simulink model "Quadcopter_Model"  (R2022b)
settings: Solver=VariableStepAuto  StartTime=0.0  StopTime=runtime  FixedStep=0.001  RelTol=1e-3
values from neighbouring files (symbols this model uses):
  delta_T = [ 0,  0,  9.404e-04 ]    [modelParameters.m]    (also in rich_params.m = [ 0,  0,  1.176e-04 ]; drone_control_system_test.m)
  g = 9.81    [modelParameters.m]    (also in rich_params.m; drone_control_system_test.m; imu_model_test.m = 0.1)
  height_controlled_o = (((Rm*If        + (((omega0_o * 2 * Rm * Kv * Kq      * Kd + 1)^2) - 1)/(4* Rm*Kv^2*Kq      * Kd))/Vb)*(Pmax - Pmin) + Pmin)    [modelParameters.m]    (also in rich_params.m)
  If = 0.3836    [modelParameters.m]    (also in rich_params.m = 0.39; drone_control_system_test.m)
  Jreq = 4.2012e-05    [modelParameters.m]    (also in rich_params.m = 1.376e-05; drone_control_system_test.m)
  Jxx = 0.0110    (= 0.011)    [modelParameters.m]    (also in rich_params.m = 0.0081; drone_control_system_test.m)
  Jyy = 0.0116    [modelParameters.m]    (also in rich_params.m = 0.0074; drone_control_system_test.m)
  Jzz = 0.0223    [modelParameters.m]    (also in rich_params.m = 0.0135; drone_control_system_test.m)
  Kd = 1.4852e-07    [modelParameters.m]    (also in rich_params.m = 5.194e-07; drone_control_system_test.m)
  Kh = 3.4574e-04    (= 0.00034574)    [modelParameters.m]    (also in rich_params.m; drone_control_system_test.m)
  Kq = 96.3422    [modelParameters.m]    (also in rich_params.m = 110; drone_control_system_test.m)
  Kt = 1.2007e-05    [modelParameters.m]    (also in rich_params.m = 7.3956e-06; drone_control_system_test.m)
  Kv = 96.3422    [modelParameters.m]    (also in rich_params.m = 110; drone_control_system_test.m)
  m = 1.216    [modelParameters.m]    (also in rich_params.m = 0.656; drone_control_system_test.m)
  omega0_o = sqrt((m*g)/(4*Kt))    [modelParameters.m]    (also in rich_params.m)
  omega1_o = sqrt((m*g)/(4*Kt))    [modelParameters.m]    (also in rich_params.m)
  omega2_o = sqrt((m*g)/(4*Kt))    [modelParameters.m]    (also in rich_params.m)
  omega3_o = sqrt((m*g)/(4*Kt))    [modelParameters.m]    (also in rich_params.m)
  pitch_o = 0    [modelParameters.m]    (also in rich_params.m)
  pitchrate_o = 0    [modelParameters.m]    (also in rich_params.m)
  Pmax = 1    [modelParameters.m]    (also in rich_params.m; drone_control_system_test.m)
  Pmin = 0    [modelParameters.m]    (also in rich_params.m; drone_control_system_test.m)
  r_oc = [ 0 ; 0 ; 0 ]    [modelParameters.m]    (also in rich_params.m; drone_control_system_test.m = [0; 0; 0]; imu_model_test.m = 0.1)
  rhx = 0.16    [modelParameters.m]    (also in rich_params.m = 0.115; drone_control_system_test.m)
  rhy = 0.16    [modelParameters.m]    (also in rich_params.m = 0.115; drone_control_system_test.m)
  rhz = 0.03    [modelParameters.m]    (also in rich_params.m = 0.04; drone_control_system_test.m)
  Rm = 0.235    [modelParameters.m]    (also in rich_params.m = 0.19; drone_control_system_test.m)
  roll_o = 0    [modelParameters.m]    (also in rich_params.m)
  rollrate_o = 0    [modelParameters.m]    (also in rich_params.m)
  signal_mixer = [ 1, -1, -1, -1    [modelParameters.m]    (also in rich_params.m; drone_control_system_test.m)
  Tc = 0.01    [modelParameters.m]    (also in rich_params.m; drone_control_system_test.m)
  Tq = 0.005    [modelParameters.m]    (also in rich_params.m; drone_control_system_test.m)
  Vb = 12.3    [modelParameters.m]    (also in rich_params.m = 11.4; drone_control_system_test.m)
  x_controlled_o = 0    [modelParameters.m]    (also in rich_params.m)
  x_o = 0    [modelParameters.m]    (also in rich_params.m)
  x_vel_o = 0    [modelParameters.m]    (also in rich_params.m)
  y_controlled_o = 0    [modelParameters.m]    (also in rich_params.m)
  y_o = 0    [modelParameters.m]    (also in rich_params.m)
  y_vel_o = 0    [modelParameters.m]    (also in rich_params.m)
  yaw_controlled_o = 0    [modelParameters.m]    (also in rich_params.m)
  yaw_o = 0    [modelParameters.m]    (also in rich_params.m)
  yawrate_o = 0    [modelParameters.m]    (also in rich_params.m)
  z_o = 0    [modelParameters.m]    (also in rich_params.m)
  z_vel_o = 0    [modelParameters.m]    (also in rich_params.m)
undefined symbols (not defined in the file or in its folder): lqr_K
libraries: Derivative x13, slpidlib x13, dsparch4 x3, vrlib x2, simulink_need_slupdate x2, simulink x1
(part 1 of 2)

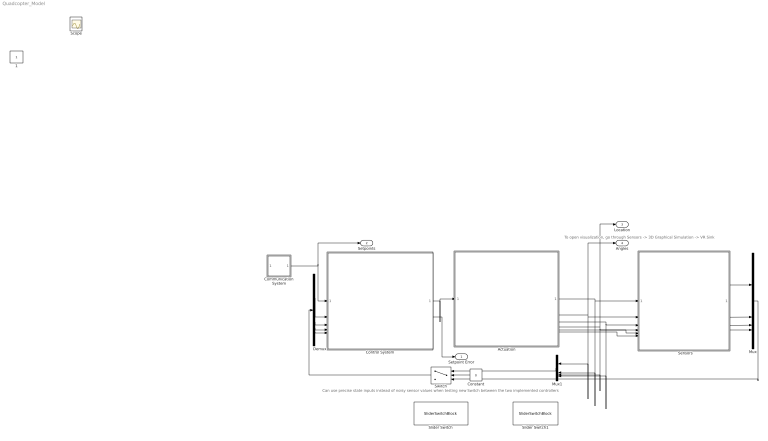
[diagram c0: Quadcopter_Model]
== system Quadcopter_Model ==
  note: To open visualization, go through Sensors -> 3D Graphical Simulation -> VR Sink
  note: Can use precise state inputs instead of noisy sensor values when testing new controls
  note: Switch between the two implemented controllers
  "     Sensors   " : Subsystem
  Actuation : Subsystem
  Communication System : Subsystem
  Constant : Constant  Value=0
  Control System : Subsystem
  Demux : Demux
  Mux : Mux
  Mux1 : Mux
  Slider Switch : SliderSwitchBlock  LabelPosition=Hide
  Slider Switch1 : SliderSwitchBlock  LabelPosition=Hide
  Switch : Switch  Criteria=u2 ~= 0
  Setpoint Error : Outport  SignalName=setpoint_error
  Setpoints : Outport  Port=2
  Location : Outport  Port=3
  Angles : Outport  Port=4
  1 : Constant  IOType=siggen
  Scope : Scope
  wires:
  Actuation/6(B_g) -> 1/6
  Actuation/5(B_vo_dot) -> 1/5
  Actuation/1(B_omega) -> Mux1/2, 1/1
  Actuation/2(euler_angles) -> 1/2, Mux1/1, Angles/1
  Communication System/1(setpoints1) -> Setpoints/1, Control System/1(setpoints)
  Actuation/3(B_vo) -> 1/3, Mux1/4
  1/2 -> Mux/2
  1/1 -> Mux/1
  1/3 -> Mux/3
  Mux/1 -> Switch/3
  Mux1/1 -> Switch/1
  Demux/4 -> Control System/5(velocity)
  Demux/3 -> Control System/4(current_position)
  Demux/2 -> Control System/3(euler_rates)
  Demux/1 -> Control System/2(euler_angles_filtered)
  Switch/1 -> Demux/1
  Constant/1 -> Switch/2
  1/4 -> Mux/4
  Actuation/4(E_ro) -> 1/4, Mux1/3, Location/1
  Control System/2(setpoint error) -> Setpoint Error/1
  Control System/1(P) -> Actuation/1(P)

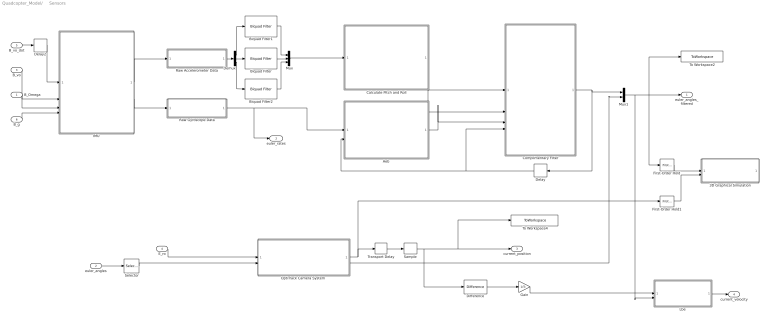
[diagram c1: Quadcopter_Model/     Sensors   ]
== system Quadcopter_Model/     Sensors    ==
  B_Omega : Inport
  euler_angles : Inport  Port=2
  B_vo : Inport  Port=3
  E_ro : Inport  Port=4
  B_vo_dot : Inport  Port=5
  B_g : Inport  Port=6
  3D Graphical Simulation : Subsystem
  "Aeb " : MATLAB Function  TreatAsAtomicUnit=on
  Biquad Filter : dsparch4/Biquad Filter  FilterSource=Dialog parameters  CoeffSource=Specify via dialog  FilterObject=BQF  IIRFiltStruct=Direct form II  BiQuadCoeffs=accel_SOS_Matrix  ScaleValues=1  IC=0  ICnum=0  ICden=0  a0Flag=Warning  optimizeScaleValues=on  ScaleValueMode=Specify via input port (g)  InputProcessing=Columns as channels (frame based)  roundingMode=Floor  overflowMode=off  scaleValueFracLength=14  denProdOutputFracLength=30  denAccumFracLength=30  secondMemoryFracLength=15
  Biquad Filter1 : dsparch4/Biquad Filter  FilterSource=Dialog parameters  CoeffSource=Specify via dialog  FilterObject=BQF  IIRFiltStruct=Direct form II  BiQuadCoeffs=accel_SOS_Matrix  ScaleValues=1  IC=0  ICnum=0  ICden=0  a0Flag=Warning  optimizeScaleValues=on  ScaleValueMode=Specify via input port (g)  InputProcessing=Columns as channels (frame based)  roundingMode=Floor  overflowMode=off  scaleValueFracLength=14  denProdOutputFracLength=30  denAccumFracLength=30  secondMemoryFracLength=15
  Biquad Filter2 : dsparch4/Biquad Filter  FilterSource=Dialog parameters  CoeffSource=Specify via dialog  FilterObject=BQF  IIRFiltStruct=Direct form II  BiQuadCoeffs=accel_SOS_Matrix  ScaleValues=1  IC=0  ICnum=0  ICden=0  a0Flag=Warning  optimizeScaleValues=on  ScaleValueMode=Specify via input port (g)  InputProcessing=Columns as channels (frame based)  roundingMode=Floor  overflowMode=off  scaleValueFracLength=14  denProdOutputFracLength=30  denAccumFracLength=30  secondMemoryFracLength=15
  Calculate Pitch and Roll : MATLAB Function  TreatAsAtomicUnit=on
  Complimentary Filter : MATLAB Function  TreatAsAtomicUnit=on
  Delay : Delay  DelayLength=1  InitialCondition=0
  Delay2 : Delay  DelayLength=1  InitialCondition=0  SampleTime=Tq
  Demux : Demux  Outputs=3
  Difference : simulink/Discrete/Difference  ICPrevInput=0.0  OutMin=[]  OutMax=[]  OutDataType=fixdt(1, 16)  OutScaling=2^-10  DoSatur=off
  First-Order Hold : simulink_need_slupdate/First-Order Hold  DisableCoverage=on  Ts=5e-3
  First-Order Hold1 : simulink_need_slupdate/First-Order Hold  DisableCoverage=on  Ts=5e-3
  Gain : Gain  Gain=1/Tc
  "IMU " : Subsystem
  "Lbe " : MATLAB Function  TreatAsAtomicUnit=on
  Mux : Mux  Inputs=3
  Mux1 : Mux  Inputs=2
  "OptiTrack Camera System " : Subsystem
  Raw Accelerometer Data : Subsystem  Variant=on
  Raw Gyroscope Data : Subsystem  Variant=on
  Sample : ZeroOrderHold  SampleTime=Tc
  Selector : Selector  InputPortWidth=3  IndexOptions=Index vector (dialog)  Indices=[3]  OutputSizes=1
  To Workspace2 : ToWorkspace  VariableName=angle_IMU_reading  SaveFormat=Structure With Time  SampleTime=Tq
  To Workspace4 : ToWorkspace  VariableName=position_model  SaveFormat=Structure With Time  SampleTime=Tc
  Transport Delay : TransportDelay  DelayTime=6e-3
  euler_angles_filtered : Outport
  euler_rates : Outport  Port=2
  current_position : Outport  Port=3
  current_velocity : Outport  Port=4
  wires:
  "IMU "/1(accelerometer) -> Raw Accelerometer Data/1(raw_accel_model)
  "IMU "/2(gyroscope) -> Raw Gyroscope Data/1(raw_gyro_model)
  B_vo/1 -> "IMU "/2(B_vo)
  B_Omega/1 -> "IMU "/3(B_Omega)
  B_g/1 -> "IMU "/4(B_g)
  Calculate Pitch and Roll/2(accel_roll) -> Complimentary Filter/2(accel_roll)
  Calculate Pitch and Roll/1(accel_pitch) -> Complimentary Filter/1(accel_pitch)
  First-Order Hold/1 -> 3D Graphical Simulation/1("Euler Angles ")
  E_ro/1 -> "OptiTrack Camera System "/1(E_ro)
  First-Order Hold1/1 -> 3D Graphical Simulation/2(Displacement)
  B_vo_dot/1 -> Delay2/1
  Delay2/1 -> "IMU "/1(B_vo_dot)
  "OptiTrack Camera System "/1(E_ro_camera) -> Transport Delay/1, First-Order Hold1/1
  Transport Delay/1 -> Sample/1
  Raw Gyroscope Data/1(raw_gyro) -> "Aeb "/1(gyro_reading), euler_rates/1
  Delay/1 -> Complimentary Filter/4(prev_euler_angles), "Aeb "/2(euler_angles_filtered)
  "OptiTrack Camera System "/2(yaw_camera) -> Mux1/2
  "Aeb "/1(euler_rates_IMU) -> Complimentary Filter/3(euler_rates_gyro)
  Raw Accelerometer Data/1(raw_accel) -> Demux/1
  Demux/2 -> Biquad Filter/1
  Demux/1 -> Biquad Filter1/1
  Demux/3 -> Biquad Filter2/1
  Biquad Filter/1 -> Mux/2
  Biquad Filter1/1 -> Mux/1
  Biquad Filter2/1 -> Mux/3
  Mux/1 -> Calculate Pitch and Roll/1(accel_reading)
  Complimentary Filter/1(euler_angles_IMU) -> Mux1/1, Delay/1
  euler_angles/1 -> Selector/1
  Selector/1 -> "OptiTrack Camera System "/2(yaw)
  Mux1/1 -> To Workspace2/1, First-Order Hold/1, euler_angles_filtered/1, "Lbe "/2(euler_angles)
  Difference/1 -> Gain/1
  Gain/1 -> "Lbe "/1(E_vo)
  "Lbe "/1(B_vo) -> current_velocity/1
  Sample/1 -> Difference/1, To Workspace4/1, current_position/1

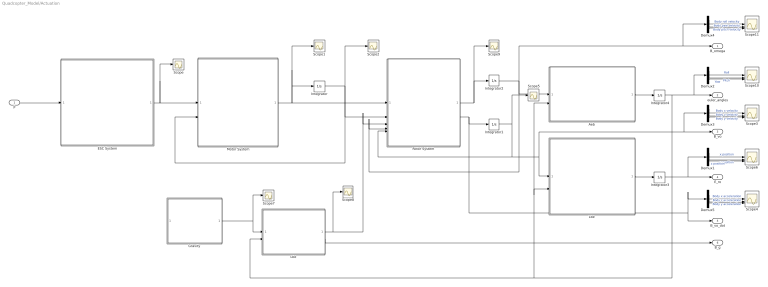
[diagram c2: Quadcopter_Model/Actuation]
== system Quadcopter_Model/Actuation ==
  P : Inport
  "Aeb " : MATLAB Function  TreatAsAtomicUnit=on
  Demux{1..5} (5 alike) : Demux  Outputs=3
  ESC System : MATLAB Function  TreatAsAtomicUnit=on
  "Gravity " : MATLAB Function  TreatAsAtomicUnit=on
  Integrator : Integrator  InitialCondition=[omega0_o, omega1_o, omega2_o, omega3_o]
  Integrator1 : Integrator  InitialCondition=[x_vel_o; y_vel_o; z_vel_o]
  Integrator2 : Integrator  InitialCondition=[rollrate_o; pitchrate_o; yawrate_o]
  Integrator3 : Integrator  InitialCondition=[x_o; y_o; z_o]
  Integrator4 : Integrator  InitialCondition=[roll_o; pitch_o; yaw_o]  ContinuousStateAttributes=['phi' 'theta' 'psi']
  "Lbe " : MATLAB Function  TreatAsAtomicUnit=on
  "Lbe " : MATLAB Function  TreatAsAtomicUnit=on
  Motor System : MATLAB Function  TreatAsAtomicUnit=on
  "Rotor System " : MATLAB Function  TreatAsAtomicUnit=on
  Scope{,1..2,5,7..9} (7 alike) : Scope
  Scope{3..4,6,10..11} (5 alike) : Scope  NumInputPorts=3
  B_omega : Outport
  euler_angles : Outport  Port=2
  B_vo : Outport  Port=3
  E_ro : Outport  Port=4
  B_vo_dot : Outport  Port=5
  B_g : Outport  Port=6
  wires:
  ESC System/1(Vb_eff) -> Scope/1, Motor System/1(Vb_eff)
  "Rotor System "/1(B_omega_dot) -> Scope9/1, Integrator2/1
  Integrator2/1 -> "Rotor System "/4(B_omega), B_omega/1, Demux4/1, "Aeb "/1(B_omega)
  "Aeb "/1(euler_rates) -> Integrator4/1
  "Lbe "/1(E_ro) -> Integrator3/1
  Integrator3/1 -> Demux1/1, E_ro/1
  "Lbe "/1(B_Fg) -> Scope8/1, "Rotor System "/3(B_Fg)
  "Lbe "/2(B_g) -> B_g/1
  Demux1/2 -> Scope6/2  "y position"
  Demux1/1 -> Scope6/1  "x position"
  Demux1/3 -> Scope6/3  "z position"
  Demux2/2 -> Scope10/2  "Pitch"
  Demux2/1 -> Scope10/1  "Roll"
  Demux2/3 -> Scope10/3  "Yaw"
  Demux4/2 -> Scope11/2  "Body pitch velocity"
  Demux4/1 -> Scope11/1  "Body roll velocity"
  Demux4/3 -> Scope11/3  "Body yaw velocity"
  Demux3/2 -> Scope3/2  "Body y velocity"
  Demux3/1 -> Scope3/1  "Body x velocity"
  Demux3/3 -> Scope3/3  "Body z velocity"
  Demux5/2 -> Scope4/2  "Body y acceleration"
  Demux5/1 -> Scope4/1  "Body x acceleration"
  Demux5/3 -> Scope4/3  "Body z acceleration"
  Integrator1/1 -> Scope5/1, "Rotor System "/5(B_vo), "Lbe "/1(B_vo), Demux3/1, B_vo/1
  "Rotor System "/2(B_vo_dot) -> Demux5/1, B_vo_dot/1, Integrator1/1
  Integrator4/1 -> euler_angles/1, Demux2/1, "Lbe "/2(euler_angles), "Aeb "/2(euler_angles), "Lbe "/2(euler_angles)
  P/1 -> ESC System/1(P)
  "Gravity "/1(E_Fg) -> Scope7/1, "Lbe "/1(E_Fg)
  Integrator/1 -> Motor System/2(w), "Rotor System "/2(w), Scope2/1
  Motor System/1(w_dot) -> Integrator/1, Scope1/1, "Rotor System "/1(w_dot)

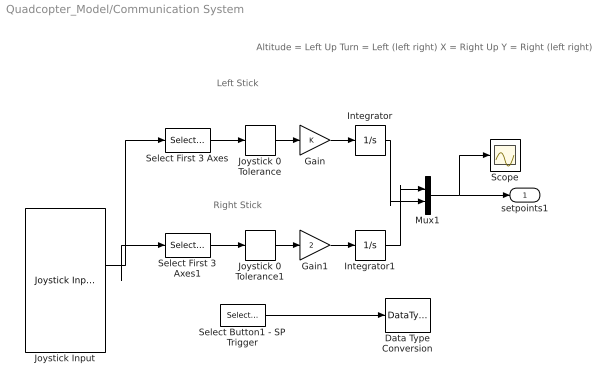
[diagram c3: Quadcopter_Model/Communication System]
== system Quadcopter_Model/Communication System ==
  note: Altitude = Left Up Turn = Left (left right) X = Right Up Y = Right (left right)
  note: Right Stick
  note: Left Stick
  Data Type Conversion : DataTypeConversion  Commented=on  OutDataTypeStr=boolean
  Gain : Gain
  Gain1 : Gain  Gain=2
  Integrator : Integrator
  Integrator1 : Integrator
  Joystick 0 Tolerance : DeadZone  LowerValue=-0.3  UpperValue=0.3
  Joystick 0 Tolerance1 : DeadZone  LowerValue=-0.3  UpperValue=0.3
  Joystick Input : vrlib/Joystick Input  joyid=1  adjustports=on  forcefeed=off
  Mux1 : Mux  Inputs=2
  Scope : Scope
  Select Button1 - SP Trigger : Selector  Commented=on  InputPortWidth=10  IndexOptions=Index vector (dialog)  Indices=[1]  OutputSizes=1
  Select First 3 Axes : Selector  InputPortWidth=5  IndexOptions=Index vector (dialog)  Indices=[2 1]  OutputSizes=1
  Select First 3 Axes1 : Selector  InputPortWidth=5  IndexOptions=Index vector (dialog)  Indices=[5 4]  OutputSizes=1
  setpoints1 : Outport
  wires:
  Gain1/1 -> Integrator1/1
  Select First 3 Axes/1 -> Joystick 0 Tolerance/1
  Joystick 0 Tolerance1/1 -> Gain1/1
  Gain/1 -> Integrator/1
  Mux1/1 -> setpoints1/1, Scope/1
  Integrator/1 -> Mux1/2
  Integrator1/1 -> Mux1/1
  Select First 3 Axes1/1 -> Joystick 0 Tolerance1/1
  Joystick 0 Tolerance/1 -> Gain/1
  Joystick Input/1 -> Select First 3 Axes1/1, Select First 3 Axes/1
  Select Button1 - SP Trigger/1 -> Data Type Conversion/1

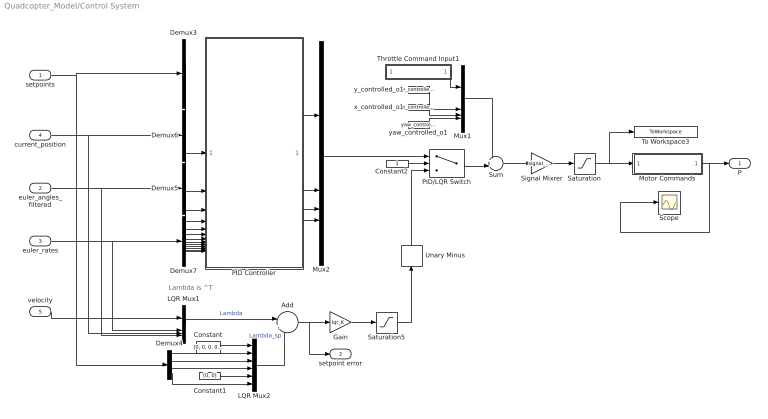
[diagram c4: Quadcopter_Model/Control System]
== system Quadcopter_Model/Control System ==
  note: Lambda is ^T
  setpoints : Inport
  euler_angles_filtered : Inport  Port=2
  euler_rates : Inport  Port=3
  current_position : Inport  Port=4
  velocity : Inport  Port=5
  Add : Sum  Inputs=|+-
  Constant : Constant  Value=[0, 0, 0, 0, 0, 0]
  Constant1 : Constant  Value=[0, 0]
  Constant2 : Constant
  Demux3 : Demux
  Demux4 : Demux
  Demux5 : Demux  Outputs=3
  Demux6 : Demux  Outputs=3
  Demux7 : Demux  Outputs=3
  Gain : Gain  Gain=lqr_K  Multiplication=Matrix(K*u)
  LQR Mux1 : Mux
  LQR Mux2 : Mux  Inputs=6
  Motor Commands : Subsystem  Variant=on
  Mux1 : Mux
  Mux2 : Mux
  PID Controller : Subsystem
  PID/LQR Switch : Switch  Criteria=u2 ~= 0
  Saturation : Saturate  UpperLimit=Pmax*ones(4,1)  LowerLimit=Pmin*ones(4,1)
  Saturation5 : Saturate  UpperLimit=[20000, 20000, 20000, 20000]  LowerLimit=[-20000, -20000, -20000, -20000]
  Scope : Scope
  Signal Mixrer : Gain  Gain=signal_mixer  Multiplication=Matrix(K*u)
  Sum : Sum  Inputs=++|
  Throttle Command Input1 : Subsystem  Variant=on
  To Workspace3 : ToWorkspace  VariableName=motorCommands  SaveFormat=Structure With Time  SampleTime=Tq
  Unary Minus : UnaryMinus
  x_controlled_o1 : Constant  Value=x_controlled_o
  y_controlled_o1 : Constant  Value=y_controlled_o
  yaw_controlled_o1 : Constant  Value=yaw_controlled_o
  P : Outport
  setpoint error : Outport  Port=2
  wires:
  Motor Commands/1(z_command) -> P/1, Scope/1
  Saturation/1 -> To Workspace3/1, Motor Commands/1(z_command_model)
  setpoints/1 -> Demux3/1, Demux4/1
  current_position/1 -> Demux6/1, LQR Mux1/3
  euler_angles_filtered/1 -> LQR Mux1/4, Demux5/1
  euler_rates/1 -> Demux7/1, LQR Mux1/2
  Demux3/1 -> PID Controller/1(x_setpoint)
  Demux3/2 -> PID Controller/2(y_setpoint)
  Demux3/3 -> PID Controller/3(z_setpoint)
  Demux3/4 -> PID Controller/4(yaw_setpoint)
  Demux6/1 -> PID Controller/5(x_position)
  Demux6/2 -> PID Controller/6(y_position)
  Demux5/2 -> PID Controller/9(pitch)
  Demux5/3 -> PID Controller/10(yaw)
  Demux7/1 -> PID Controller/11(roll_rate)
  Demux7/2 -> PID Controller/12(pitch_rate)
  PID Controller/1(height_controlled) -> Mux2/1
  PID Controller/2(y_controlled) -> Mux2/2
  PID Controller/3(x_controlled) -> Mux2/3
  PID Controller/4(yaw_controlled) -> Mux2/4
  Mux2/1 -> PID/LQR Switch/1
  Demux4/1 -> LQR Mux2/2
  Demux4/2 -> LQR Mux2/3
  Demux4/3 -> LQR Mux2/4
  Demux4/4 -> LQR Mux2/6
  Constant/1 -> LQR Mux2/1
  Constant1/1 -> LQR Mux2/5
  LQR Mux1/1 -> Add/1  "Lambda"
  LQR Mux2/1 -> Add/2  "Lambda_sp"
  Demux7/3 -> PID Controller/13(yaw_rate)
  Demux5/1 -> PID Controller/8(roll)
  Demux6/3 -> PID Controller/7(z_position)
  Gain/1 -> Saturation5/1
  Saturation5/1 -> Unary Minus/1
  Unary Minus/1 -> PID/LQR Switch/3
  yaw_controlled_o1/1 -> Mux1/4
  x_controlled_o1/1 -> Mux1/3
  y_controlled_o1/1 -> Mux1/2
  Throttle Command Input1/1(z_command) -> Mux1/1
  PID/LQR Switch/1 -> Sum/2
  Signal Mixrer/1 -> Saturation/1
  Sum/1 -> Signal Mixrer/1
  Mux1/1 -> Sum/1
  Constant2/1 -> PID/LQR Switch/2
  Add/1 -> setpoint error/1, Gain/1
  velocity/1 -> LQR Mux1/1

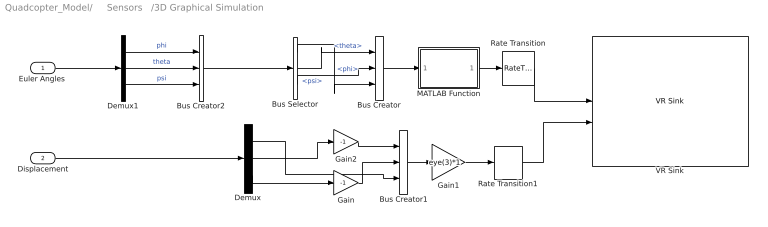
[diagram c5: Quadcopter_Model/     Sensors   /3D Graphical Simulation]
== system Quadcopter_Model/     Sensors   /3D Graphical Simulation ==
  "Euler Angles " : Inport
  Displacement : Inport  Port=2
  Bus Creator : BusCreator  Inputs=3
  Bus Creator1 : BusCreator  Inputs=3
  Bus Creator2 : BusCreator  Inputs=3
  Bus Selector : BusSelector  OutputSignals=phi,theta,psi
  Demux : Demux  Outputs=3
  Demux1 : Demux  Outputs=3
  Gain : Gain  Gain=-1
  Gain1 : Gain  Gain=eye(3)*1  Multiplication=Matrix(K*u)
  Gain2 : Gain  Gain=-1
  MATLAB Function : MATLAB Function  TreatAsAtomicUnit=on
  Rate Transition : RateTransition  OutPortSampleTime=0.06
  Rate Transition1 : RateTransition  OutPortSampleTime=0.06
  VR Sink : vrlib/VR Sink  InstantiateOnLoad=on  SampleTime=-1  ViewEnable=on  RemoteChange=off  RemoteView=off  FieldsWritten=Helicopter.rotation.4.1.1.double#Helicopter.translation.3.1.1.double  WorldFileName=quadrotor_world_ucart.wrl  AutoView=on  VideoDimensions=[]  AllowVariableSize=off
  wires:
  Bus Creator2/1 -> Bus Selector/1
  Demux/1 -> Bus Creator1/3
  Gain/1 -> Bus Creator1/2
  Gain2/1 -> Bus Creator1/1
  Rate Transition1/1 -> VR Sink/2
  Rate Transition/1 -> VR Sink/1
  Demux/3 -> Gain/1
  Demux/2 -> Gain2/1
  Bus Creator1/1 -> Gain1/1
  Bus Selector/1 -> Bus Creator/3  "<phi>"
  Bus Selector/3 -> Bus Creator/2  "<psi>"
  Bus Selector/2 -> Bus Creator/1  "<theta>"
  Gain1/1 -> Rate Transition1/1
  Demux1/3 -> Bus Creator2/3  "psi"
  Demux1/2 -> Bus Creator2/2  "theta"
  Demux1/1 -> Bus Creator2/1  "phi"
  Bus Creator/1 -> MATLAB Function/1(u)
  MATLAB Function/1(y) -> Rate Transition/1
  Displacement/1 -> Demux/1
  "Euler Angles "/1 -> Demux1/1

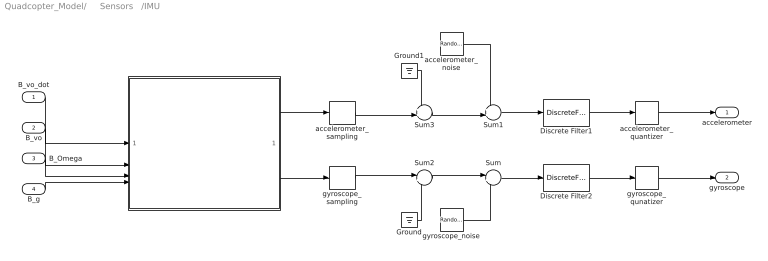
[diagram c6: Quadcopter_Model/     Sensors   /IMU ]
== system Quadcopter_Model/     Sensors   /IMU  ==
  B_vo_dot : Inport
  B_vo : Inport  Port=2
  B_Omega : Inport  Port=3
  B_g : Inport  Port=4
  " " : MATLAB Function  TreatAsAtomicUnit=on
  Discrete Filter1 : DiscreteFilter  Numerator=[0 0.749]  Denominator=[1 -0.251]  InitialStates=[0, 0, -1]  SampleTime=Tq
  Discrete Filter2 : DiscreteFilter  Numerator=[0 0.7327]  Denominator=[1 -0.2673]  SampleTime=Tq
  Ground : Ground
  Ground1 : Ground
  Sum : Sum  Inputs=|++
  Sum1 : Sum  Inputs=++|
  Sum2 : Sum  Inputs=|++
  Sum3 : Sum  Inputs=++|
  accelerometer_noise : RandomNumber  Mean=zeros(3,1)  Variance=[ 3e-7 ; 3.3e-7 ; 7.2e-7 ]  Seed=[0,1,2]  SampleTime=Tq
  accelerometer_quantizer : Quantizer  QuantizationInterval=2.4400e-04
  accelerometer_sampling : ZeroOrderHold  SampleTime=Tq
  gyroscope_noise : RandomNumber  Mean=zeros(3,1)  Variance=[ 2.2e-8 ; 1.1e-7 ; 2.4e-8 ]  Seed=[0,1,2]  SampleTime=Tq
  gyroscope_qunatizer : Quantizer  QuantizationInterval=1.1e-3
  gyroscope_sampling : ZeroOrderHold  SampleTime=Tq
  accelerometer : Outport
  gyroscope : Outport  Port=2
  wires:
  accelerometer_noise/1 -> Sum1/1
  Sum2/1 -> Sum/1
  Sum3/1 -> Sum1/2
  gyroscope_noise/1 -> Sum/2
  gyroscope_sampling/1 -> Sum2/1
  accelerometer_sampling/1 -> Sum3/2
  Ground/1 -> Sum2/2
  Ground1/1 -> Sum3/1
  B_vo_dot/1 -> " "/1(B_vo_dot)
  B_vo/1 -> " "/2(B_vo)
  B_Omega/1 -> " "/3(B_Omega)
  B_g/1 -> " "/4(B_g)
  " "/2(gyroReading) -> gyroscope_sampling/1
  " "/1(accelReading) -> accelerometer_sampling/1
  Sum1/1 -> Discrete Filter1/1
  Sum/1 -> Discrete Filter2/1
  accelerometer_quantizer/1 -> accelerometer/1
  gyroscope_qunatizer/1 -> gyroscope/1
  Discrete Filter1/1 -> accelerometer_quantizer/1
  Discrete Filter2/1 -> gyroscope_qunatizer/1

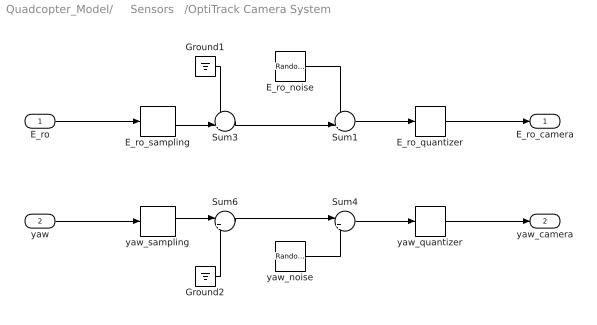
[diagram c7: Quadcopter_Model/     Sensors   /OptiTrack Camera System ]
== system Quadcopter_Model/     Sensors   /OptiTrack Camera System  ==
  E_ro : Inport
  yaw : Inport  Port=2
  E_ro_noise : RandomNumber  Mean=zeros(3,1)  Variance=[ 7.9664e-10 ; 1.1928e-10 ; 5.0636e-10 ]  Seed=[0,1,2]  SampleTime=Tc
  E_ro_quantizer : Quantizer  QuantizationInterval=2.4400e-04
  E_ro_sampling : ZeroOrderHold  SampleTime=Tc
  Ground1 : Ground
  Ground2 : Ground
  Sum1 : Sum  Inputs=++|
  Sum3 : Sum  Inputs=++|
  Sum4 : Sum  Inputs=|++
  Sum6 : Sum  Inputs=|++
  yaw_noise : RandomNumber  Variance=1.0783e-9  SampleTime=Tq
  yaw_quantizer : Quantizer  QuantizationInterval=1.1e-3
  yaw_sampling : ZeroOrderHold  SampleTime=Tq
  E_ro_camera : Outport
  yaw_camera : Outport  Port=2
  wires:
  E_ro_noise/1 -> Sum1/1
  Sum3/1 -> Sum1/2
  Sum1/1 -> E_ro_quantizer/1
  E_ro_sampling/1 -> Sum3/2
  Ground1/1 -> Sum3/1
  Sum4/1 -> yaw_quantizer/1
  Sum6/1 -> Sum4/1
  yaw_noise/1 -> Sum4/2
  yaw_sampling/1 -> Sum6/1
  Ground2/1 -> Sum6/2
  yaw/1 -> yaw_sampling/1
  E_ro/1 -> E_ro_sampling/1
  E_ro_quantizer/1 -> E_ro_camera/1
  yaw_quantizer/1 -> yaw_camera/1

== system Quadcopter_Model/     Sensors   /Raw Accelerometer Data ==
  note: 1) Add Subsystem or Model blocks as valid variant choices. 2) You cannot connect blocks at this level. At simulation, connectivity is automatically determined, based on the active variant and port name matching.
  raw_accel_model : Inport
  Feedback : Subsystem  VariantControl=logAnalysisToggle==0
  "Raw Accelerometer Data " : Subsystem  VariantControl=logAnalysisToggle==1
  raw_accel : Outport

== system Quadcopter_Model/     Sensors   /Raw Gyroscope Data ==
  note: 1) Add Subsystem or Model blocks as valid variant choices. 2) You cannot connect blocks at this level. At simulation, connectivity is automatically determined, based on the active variant and port name matching.
  raw_gyro_model : Inport
  Feedback : Subsystem  VariantControl=logAnalysisToggle==0
  "Raw Gyroscope Data " : Subsystem  VariantControl=logAnalysisToggle==1
  raw_gyro : Outport

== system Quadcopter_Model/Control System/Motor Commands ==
  note: 1) Add Subsystem or Model blocks as valid variant choices. 2) You cannot connect blocks at this level. At simulation, connectivity is automatically determined, based on the active variant and port name matching.
  z_command_model : Inport
  Feedback : Subsystem  VariantControl=logAnalysisToggle==0
  Motor Command : Subsystem  VariantControl=logAnalysisToggle==1
  z_command : Outport

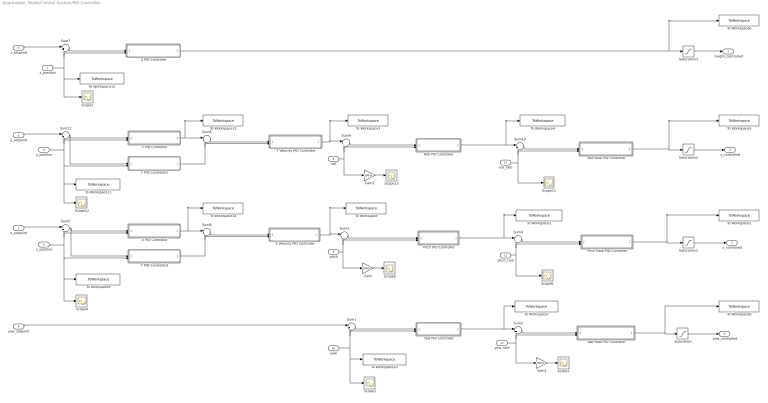
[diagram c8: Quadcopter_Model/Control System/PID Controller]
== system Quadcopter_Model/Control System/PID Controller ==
  x_setpoint : Inport
  y_setpoint : Inport  Port=2
  z_setpoint : Inport  Port=3
  yaw_setpoint : Inport  Port=4
  x_position : Inport  Port=5
  y_position : Inport  Port=6
  z_position : Inport  Port=7
  roll : Inport  Port=8
  pitch : Inport  Port=9
  yaw : Inport  Port=10
  roll_rate : Inport  Port=11
  pitch_rate : Inport  Port=12
  yaw_rate : Inport  Port=13
  Gain : Gain  Gain=180/pi
  Gain1 : Gain  Gain=180/pi
  Gain2 : Gain  Gain=180/pi
  Pitch PID Controller : Subsystem  mask{Kp=35, Ki=0, Kd=1, a=0.88, Ts=Tq}
      mask prompts: a "alpha"; Ts "Sample Time"
  Pitch Rate PID Controller : Subsystem  mask{Kp=0.03, Ki=0, Kd=0.005, a=0.88, Ts=Tq}
      mask prompts: a "alpha"; Ts "Sample Time"
  Roll PID Controller : Subsystem  mask{Kp=35, Ki=0, Kd=1, a=0.88, Ts=Tq}
      mask prompts: a "alpha"; Ts "Sample Time"
  Roll Rate PID Controller : Subsystem  mask{Kp=0.03, Ki=0, Kd=0.005, a=0.88, Ts=Tq}
      mask prompts: a "alpha"; Ts "Sample Time"
  Saturation{,1..3} (4 alike) : Saturate  UpperLimit=20000  LowerLimit=-20000
  Scope{1..4,6,9,11..13} (9 alike) : Scope
  Sum{1..11} (11 alike) : Sum  Inputs=|+-
  To Workspace : ToWorkspace  VariableName=pitch_setpoint_model  SaveFormat=Structure With Time  SampleTime=-1
  To Workspace1 : ToWorkspace  VariableName=pitchrate_setpoint_model  SaveFormat=Structure With Time  SampleTime=Tq
  To Workspace10 : ToWorkspace  VariableName=yaw_value_model  SaveFormat=Structure With Time  SampleTime=Tc
  To Workspace11 : ToWorkspace  VariableName=y_position_model  SaveFormat=Structure With Time  SampleTime=Tc
  To Workspace12 : ToWorkspace  VariableName=z_position_model  SaveFormat=Structure With Time  SampleTime=Tc
  To Workspace13 : ToWorkspace  VariableName=y_vel_setpoint_model  SaveFormat=Structure With Time  SampleTime=Tc
  To Workspace14 : ToWorkspace  VariableName=x_vel_setpoint_model  SaveFormat=Structure With Time  SampleTime=Tc
  To Workspace2 : ToWorkspace  VariableName=x_command_model  SaveFormat=Structure With Time  SampleTime=Tq
  To Workspace3 : ToWorkspace  VariableName=roll_setpoint_model  SaveFormat=Structure With Time  SampleTime=Tc
  To Workspace4 : ToWorkspace  VariableName=rollrate_setpoint_model  SaveFormat=Structure With Time  SampleTime=Tq
  To Workspace5 : ToWorkspace  VariableName=y_command_model  SaveFormat=Structure With Time  SampleTime=Tq
  To Workspace6 : ToWorkspace  VariableName=z_command_model  SaveFormat=Structure With Time  SampleTime=Tc
  To Workspace7 : ToWorkspace  VariableName=yawrate_setpoint_model  SaveFormat=Structure With Time  SampleTime=Tc
  To Workspace8 : ToWorkspace  VariableName=yaw_command_model  SaveFormat=Structure With Time  SampleTime=Tq
  To Workspace9 : ToWorkspace  VariableName=x_position_model  SaveFormat=Structure With Time  SampleTime=Tc
  X PID Controller : Subsystem  mask{Kp=0.55, Ki=0.0075, Kd=0, a=0.88, Ts=Tc}
      mask prompts: a "alpha"; Ts "Sample Time"
  X Velocity PID Controller : Subsystem  mask{Kp=-0.1, Ki=0, Kd=-0.02, a=0.00, Ts=Tc}
      mask prompts: a "alpha"; Ts "Sample Time"
  Y PID Controller : Subsystem  mask{Kp=0.55, Ki=0.0075, Kd=0, a=0.88, Ts=Tc}
      mask prompts: a "alpha"; Ts "Sample Time"
  Y PID Controller1 : Subsystem  mask{Kp=0, Ki=0, Kd=-1, a=0.88, Ts=Tc}
      mask prompts: a "alpha"; Ts "Sample Time"
  Y PID Controller2 : Subsystem  mask{Kp=0, Ki=0, Kd=-1, a=0.88, Ts=Tc}
      mask prompts: a "alpha"; Ts "Sample Time"
  Y Velocity PID Controller : Subsystem  mask{Kp=0.1, Ki=0, Kd=0.02, a=0.00, Ts=Tc}
      mask prompts: a "alpha"; Ts "Sample Time"
  Yaw PID Controller : Subsystem  mask{Kp=2.6, Ki=0, Kd=0, a=0.88, Ts=Tc}
      mask prompts: a "alpha"; Ts "Sample Time"
  Yaw Rate PID Controller : Subsystem  mask{Kp=0.297, Ki=0, Kd=0, a=0.88, Ts=Tq}
      mask prompts: a "alpha"; Ts "Sample Time"
  Z PID Controller : Subsystem  mask{Kp=-0.098040, Ki=-0.00817, Kd=-0.07353, a=0.88, Ts=Tc}
      mask prompts: a "alpha"; Ts "Sample Time"
  height_controlled : Outport
  y_controlled : Outport  Port=2
  x_controlled : Outport  Port=3
  yaw_controlled : Outport  Port=4
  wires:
  z_setpoint/1 -> Sum7/1
  Pitch PID Controller/1(pitchrate_setpoint) -> Sum4/1, To Workspace1/1
  Gain/1 -> Scope9/1
  Yaw Rate PID Controller/1(yaw_motor_command) -> To Workspace8/1, Saturation/1
  Pitch Rate PID Controller/1(x_motor_command) -> Saturation1/1, To Workspace2/1
  x_setpoint/1 -> Sum5/1
  Roll PID Controller/1(rollrate_setpoint) -> Sum10/1, To Workspace4/1
  Gain2/1 -> Scope13/1
  y_setpoint/1 -> Sum11/1
  yaw_setpoint/1 -> Sum1/1
  Gain1/1 -> Scope1/1
  Yaw PID Controller/1(yawrate_setpoint) -> Sum2/1, To Workspace7/1
  Roll Rate PID Controller/1(y_motor_command) -> To Workspace5/1, Saturation2/1
  Saturation3/1 -> height_controlled/1
  Saturation2/1 -> y_controlled/1
  Saturation1/1 -> x_controlled/1
  Saturation/1 -> yaw_controlled/1
  y_position/1 -> Y PID Controller/2(y_pos), Sum11/2, Y PID Controller1/2(y_pos), To Workspace11/1, Scope12/1
  Sum11/1 -> Y PID Controller/1(y_error), Y PID Controller1/1(y_error)
  Sum5/1 -> X PID Controller/1(x_error), Y PID Controller2/1(x_error)
  x_position/1 -> X PID Controller/2(x_pos), Sum5/2, Scope4/1, To Workspace9/1, Y PID Controller2/2(x_pos)
  Sum1/1 -> Yaw PID Controller/1(yaw_error)
  yaw/1 -> Yaw PID Controller/2(yaw_angle), Sum1/2, Scope3/1, To Workspace10/1
  Sum7/1 -> Z PID Controller/1(z_error)
  z_position/1 -> Z PID Controller/2(z_pos), Sum7/2, To Workspace12/1, Scope2/1
  Sum3/1 -> Pitch PID Controller/1(pitch_error)
  pitch/1 -> Pitch PID Controller/2(pitch_angle), Sum3/2, Gain/1
  Sum2/1 -> Yaw Rate PID Controller/1(yawrate_error)
  yaw_rate/1 -> Yaw Rate PID Controller/2(yawrate), Sum2/2, Gain1/1
  Sum4/1 -> Pitch Rate PID Controller/1(pitchrate_error)
  pitch_rate/1 -> Pitch Rate PID Controller/2(pitchrate), Sum4/2, Scope6/1
  Sum9/1 -> Roll PID Controller/1(roll_error)
  roll/1 -> Roll PID Controller/2(roll_angle), Sum9/2, Gain2/1
  Sum10/1 -> Roll Rate PID Controller/1(rollrate_error)
  roll_rate/1 -> Roll Rate PID Controller/2(rollrate), Sum10/2, Scope11/1
  Y PID Controller/1(roll_setpoint) -> To Workspace13/1, Sum6/1
  Sum6/1 -> Y Velocity PID Controller/1(y_error)
  Y PID Controller1/1(y_vel_setpoint) -> Y Velocity PID Controller/2(y_pos), Sum6/2
  X PID Controller/1(pitch_setpoint) -> To Workspace14/1, Sum8/1
  Sum8/1 -> X Velocity PID Controller/1(x_vel_error)
  Y PID Controller2/1(x_vel_setpoint) -> X Velocity PID Controller/2(x_vel), Sum8/2
  Z PID Controller/1(z_motor_command) -> To Workspace6/1, Saturation3/1
  Y Velocity PID Controller/1(roll_setpoint) -> To Workspace3/1, Sum9/1
  X Velocity PID Controller/1(pitch_setpoint) -> To Workspace/1, Sum3/1

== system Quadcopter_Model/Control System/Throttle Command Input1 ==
  note: 1) Add Subsystem or Model blocks as valid variant choices. 2) You cannot connect blocks at this level. At simulation, connectivity is automatically determined, based on the active variant and port name matching.
  Auto Takeoff : Subsystem  VariantControl=logAnalysisToggle==1
  height_controlled_o : Subsystem  VariantControl=logAnalysisToggle==0
  z_command : Outport

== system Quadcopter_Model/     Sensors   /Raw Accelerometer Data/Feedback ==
  raw_accel_model : Inport
  raw_accel : Outport
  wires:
  raw_accel_model/1 -> raw_accel/1

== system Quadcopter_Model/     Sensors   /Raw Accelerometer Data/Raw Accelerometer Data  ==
  From Workspace5 : FromWorkspace  VariableName=raw_accel_data  SampleTime=Tq
  raw_accel : Outport
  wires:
  From Workspace5/1 -> raw_accel/1

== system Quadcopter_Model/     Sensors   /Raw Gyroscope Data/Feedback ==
  raw_gyro_model : Inport
  raw_gyro : Outport
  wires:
  raw_gyro_model/1 -> raw_gyro/1

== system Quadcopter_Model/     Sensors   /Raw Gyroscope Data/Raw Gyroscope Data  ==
  From Workspace5 : FromWorkspace  VariableName=raw_gyro_data  SampleTime=Tq
  raw_gyro : Outport
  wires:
  From Workspace5/1 -> raw_gyro/1

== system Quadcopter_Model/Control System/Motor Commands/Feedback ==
  z_command_model : Inport
  z_command : Outport
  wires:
  z_command_model/1 -> z_command/1

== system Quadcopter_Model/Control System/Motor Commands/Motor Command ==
  From Workspace5 : FromWorkspace  VariableName=motor_commands  SampleTime=Tq
  z_command : Outport
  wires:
  From Workspace5/1 -> z_command/1

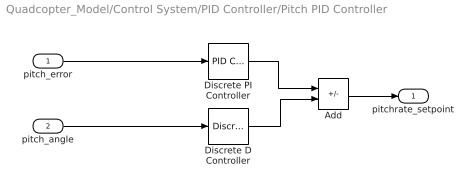
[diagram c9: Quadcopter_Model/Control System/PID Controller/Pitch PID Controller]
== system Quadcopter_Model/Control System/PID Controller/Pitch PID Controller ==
  pitch_error : Inport
  pitch_angle : Inport  Port=2
  Add : Sum  Inputs=+-
  Discrete D Controller : Derivative/Discrete D Controller  Kd=Kd  a=a
  Discrete PI Controller : slpidlib/PID Controller  Controller=PI  Form=Parallel  TimeDomain=Discrete-time  UseExternalTs=off  SampleTime=Ts  IntegratorMethod=Forward Euler  FilterMethod=Forward Euler  ControllerParametersSource=internal  P=Kp  I=Ki  UseKiTs=off  D=0  N=100  UseFilter=on  TunerSelectOption=Transfer Function Based (PID Tuner App)  InitialConditionSource=internal  InitialConditionForIntegrator=0  InitialConditionForFilter=0  DifferentiatorICPrevScaledInput=0  ExternalReset=none  TrackingMode=off  Kt=1  LimitOutput=off  SatLimitsSource=internal  UpperSaturationLimit=inf  LowerSaturationLimit=-inf  LinearizeAsGain=off  AntiWindupMode=none  Kb=1  LimitIntegrator=off  UpperIntegratorSaturationLimit=inf  LowerIntegratorSaturationLimit=-inf  POutMin=[]  POutMax=[]  IOutMin=[]  IOutMax=[]  DOutMin=[]  DOutMax=[]  NOutMin=[]  NOutMax=[]  SumOutMin=[]  SumOutMax=[]  SaturationOutMin=[]  SaturationOutMax=[]  PParamMin=[]  PParamMax=[]  IParamMin=[]  IParamMax=[]  DParamMin=[]  DParamMax=[]  NParamMin=[]  NParamMax=[]  KbParamMin=[]  KbParamMax=[]  KtParamMin=[]  KtParamMax=[]  KbOutMin=[]  KbOutMax=[]  KtOutMin=[]  KtOutMax=[]  IntegratorOutMin=[]  IntegratorOutMax=[]  FilterOutMin=[]  FilterOutMax=[]  SumI1OutMin=[]  SumI1OutMax=[]  SumI2OutMin=[]  SumI2OutMax=[]  SumI3OutMin=[]  SumI3OutMax=[]  SumI4OutMin=[]  SumI4OutMax=[]  SumDOutMin=[]  SumDOutMax=[]  DifferentiatorOutMin=[]  DifferentiatorOutMax=[]  FilterDiffOutCoefMin=[]  FilterDiffOutCoefMax=[]  ReciprocalOutMin=[]  ReciprocalOutMax=[]  SumDenOutMin=[]  SumDenOutMax=[]  SumNumOutMin=[]  SumNumOutMax=[]  DivideOutMin=[]  DivideOutMax=[]  UdiffTsProdOutMin=[]  UdiffTsProdOutMax=[]  NTsProdOutMin=[]  NTsProdOutMax=[]  UintegralTsProdOutMin=[]  UintegralTsProdOutMax=[]  UngainTsProdOutMin=[]  UngainTsProdOutMax=[]  ClampingZeroOutDataTypeStr=Inherit: Inherit via back propagation  ClampingZeroOutMin=[]  ClampingZeroOutMax=[]  FilterDenConstantOutDataTypeStr=Inherit: Inherit via back propagation  FilterDenConstantOutMin=[]  FilterDenConstantOutMax=[]  PCopyOutDataTypeStr=Inherit: Inherit via back propagation  PCopyOutMin=[]  PCopyOutMax=[]  NCopyOutDataTypeStr=Inherit: Inherit via back propagation  NCopyOutMin=[]  NCopyOutMax=[]  IntegratorContinuousStateAttributes=''  IntegratorStateMustResolveToSignalObject=off  IntegratorRTWStateStorageClass=Auto  FilterContinuousStateAttributes=''  FilterStateMustResolveToSignalObject=off  FilterRTWStateStorageClass=Auto  ParallelPVariant=InternalParameters  IdealPVariant=Disabled  IVariant=InternalParameters  DVariant=Disabled  IntegratorVariant=Discrete  SatVariant=Disabled  AWVariant=Passthrough  PCopyVariant=Disabled  TRVariant=Disabled  FdbkBlocksVariant=Forward  IdealPFdbkVariant=Disabled  SatFdbkVariant=Disabled  DerivativeFilterVariant=Disabled  NVariant=Disabled  NCopyVariant=Disabled_SignalSpec  FilterICVariant=Disabled  IntegratorICVariant=InternalICs  ExternalResetVariant=Disabled  TRSumVariant=Passthrough  SumFdbkVariant=Disabled  SumVariant=Sum_PI  TsampFilterVariant=InternalTs  TsampNgainVariant=Passthrough  TsampIntegralVariant=Passthrough  ExternalSaturationOutDataTypeStr=Inherit: Same as second input  InitialConditionSetting=Output
  pitchrate_setpoint : Outport
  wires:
  pitch_angle/1 -> Discrete D Controller/1
  pitch_error/1 -> Discrete PI Controller/1
  Discrete PI Controller/1 -> Add/1
  Discrete D Controller/1 -> Add/2
  Add/1 -> pitchrate_setpoint/1

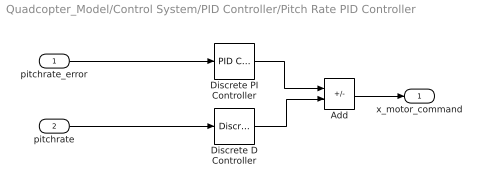
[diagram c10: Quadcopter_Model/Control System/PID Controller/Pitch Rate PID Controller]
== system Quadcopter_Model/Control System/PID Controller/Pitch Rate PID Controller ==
  pitchrate_error : Inport
  pitchrate : Inport  Port=2
  Add : Sum  Inputs=+-
  Discrete D Controller : Derivative/Discrete D Controller  Kd=Kd  a=a
  Discrete PI Controller : slpidlib/PID Controller  Controller=PI  Form=Parallel  TimeDomain=Discrete-time  UseExternalTs=off  SampleTime=Ts  IntegratorMethod=Forward Euler  FilterMethod=Forward Euler  ControllerParametersSource=internal  P=Kp  I=Ki  UseKiTs=off  D=0  N=100  UseFilter=on  TunerSelectOption=Transfer Function Based (PID Tuner App)  InitialConditionSource=internal  InitialConditionForIntegrator=0  InitialConditionForFilter=0  DifferentiatorICPrevScaledInput=0  ExternalReset=none  TrackingMode=off  Kt=1  LimitOutput=off  SatLimitsSource=internal  UpperSaturationLimit=inf  LowerSaturationLimit=-inf  LinearizeAsGain=off  AntiWindupMode=none  Kb=1  LimitIntegrator=off  UpperIntegratorSaturationLimit=inf  LowerIntegratorSaturationLimit=-inf  POutMin=[]  POutMax=[]  IOutMin=[]  IOutMax=[]  DOutMin=[]  DOutMax=[]  NOutMin=[]  NOutMax=[]  SumOutMin=[]  SumOutMax=[]  SaturationOutMin=[]  SaturationOutMax=[]  PParamMin=[]  PParamMax=[]  IParamMin=[]  IParamMax=[]  DParamMin=[]  DParamMax=[]  NParamMin=[]  NParamMax=[]  KbParamMin=[]  KbParamMax=[]  KtParamMin=[]  KtParamMax=[]  KbOutMin=[]  KbOutMax=[]  KtOutMin=[]  KtOutMax=[]  IntegratorOutMin=[]  IntegratorOutMax=[]  FilterOutMin=[]  FilterOutMax=[]  SumI1OutMin=[]  SumI1OutMax=[]  SumI2OutMin=[]  SumI2OutMax=[]  SumI3OutMin=[]  SumI3OutMax=[]  SumI4OutMin=[]  SumI4OutMax=[]  SumDOutMin=[]  SumDOutMax=[]  DifferentiatorOutMin=[]  DifferentiatorOutMax=[]  FilterDiffOutCoefMin=[]  FilterDiffOutCoefMax=[]  ReciprocalOutMin=[]  ReciprocalOutMax=[]  SumDenOutMin=[]  SumDenOutMax=[]  SumNumOutMin=[]  SumNumOutMax=[]  DivideOutMin=[]  DivideOutMax=[]  UdiffTsProdOutMin=[]  UdiffTsProdOutMax=[]  NTsProdOutMin=[]  NTsProdOutMax=[]  UintegralTsProdOutMin=[]  UintegralTsProdOutMax=[]  UngainTsProdOutMin=[]  UngainTsProdOutMax=[]  ClampingZeroOutDataTypeStr=Inherit: Inherit via back propagation  ClampingZeroOutMin=[]  ClampingZeroOutMax=[]  FilterDenConstantOutDataTypeStr=Inherit: Inherit via back propagation  FilterDenConstantOutMin=[]  FilterDenConstantOutMax=[]  PCopyOutDataTypeStr=Inherit: Inherit via back propagation  PCopyOutMin=[]  PCopyOutMax=[]  NCopyOutDataTypeStr=Inherit: Inherit via back propagation  NCopyOutMin=[]  NCopyOutMax=[]  IntegratorContinuousStateAttributes=''  IntegratorStateMustResolveToSignalObject=off  IntegratorRTWStateStorageClass=Auto  FilterContinuousStateAttributes=''  FilterStateMustResolveToSignalObject=off  FilterRTWStateStorageClass=Auto  ParallelPVariant=InternalParameters  IdealPVariant=Disabled  IVariant=InternalParameters  DVariant=Disabled  IntegratorVariant=Discrete  SatVariant=Disabled  AWVariant=Passthrough  PCopyVariant=Disabled  TRVariant=Disabled  FdbkBlocksVariant=Forward  IdealPFdbkVariant=Disabled  SatFdbkVariant=Disabled  DerivativeFilterVariant=Disabled  NVariant=Disabled  NCopyVariant=Disabled_SignalSpec  FilterICVariant=Disabled  IntegratorICVariant=InternalICs  ExternalResetVariant=Disabled  TRSumVariant=Passthrough  SumFdbkVariant=Disabled  SumVariant=Sum_PI  TsampFilterVariant=InternalTs  TsampNgainVariant=Passthrough  TsampIntegralVariant=Passthrough  ExternalSaturationOutDataTypeStr=Inherit: Same as second input
  x_motor_command : Outport
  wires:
  pitchrate/1 -> Discrete D Controller/1
  pitchrate_error/1 -> Discrete PI Controller/1
  Discrete PI Controller/1 -> Add/1
  Discrete D Controller/1 -> Add/2
  Add/1 -> x_motor_command/1

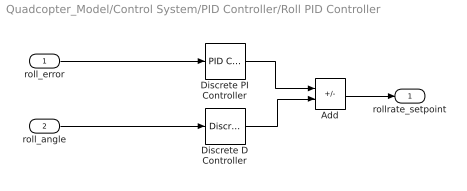
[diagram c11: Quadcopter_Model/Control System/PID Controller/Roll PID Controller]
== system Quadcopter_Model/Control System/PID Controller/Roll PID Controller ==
  roll_error : Inport
  roll_angle : Inport  Port=2
  Add : Sum  Inputs=+-
  Discrete D Controller : Derivative/Discrete D Controller  Kd=Kd  a=a
  Discrete PI Controller : slpidlib/PID Controller  Controller=PI  Form=Parallel  TimeDomain=Discrete-time  UseExternalTs=off  SampleTime=Ts  IntegratorMethod=Forward Euler  FilterMethod=Forward Euler  ControllerParametersSource=internal  P=Kp  I=Ki  UseKiTs=off  D=0  N=100  UseFilter=on  TunerSelectOption=Transfer Function Based (PID Tuner App)  InitialConditionSource=internal  InitialConditionForIntegrator=0  InitialConditionForFilter=0  DifferentiatorICPrevScaledInput=0  ExternalReset=none  TrackingMode=off  Kt=1  LimitOutput=off  SatLimitsSource=internal  UpperSaturationLimit=inf  LowerSaturationLimit=-inf  LinearizeAsGain=off  AntiWindupMode=none  Kb=1  LimitIntegrator=off  UpperIntegratorSaturationLimit=inf  LowerIntegratorSaturationLimit=-inf  POutMin=[]  POutMax=[]  IOutMin=[]  IOutMax=[]  DOutMin=[]  DOutMax=[]  NOutMin=[]  NOutMax=[]  SumOutMin=[]  SumOutMax=[]  SaturationOutMin=[]  SaturationOutMax=[]  PParamMin=[]  PParamMax=[]  IParamMin=[]  IParamMax=[]  DParamMin=[]  DParamMax=[]  NParamMin=[]  NParamMax=[]  KbParamMin=[]  KbParamMax=[]  KtParamMin=[]  KtParamMax=[]  KbOutMin=[]  KbOutMax=[]  KtOutMin=[]  KtOutMax=[]  IntegratorOutMin=[]  IntegratorOutMax=[]  FilterOutMin=[]  FilterOutMax=[]  SumI1OutMin=[]  SumI1OutMax=[]  SumI2OutMin=[]  SumI2OutMax=[]  SumI3OutMin=[]  SumI3OutMax=[]  SumI4OutMin=[]  SumI4OutMax=[]  SumDOutMin=[]  SumDOutMax=[]  DifferentiatorOutMin=[]  DifferentiatorOutMax=[]  FilterDiffOutCoefMin=[]  FilterDiffOutCoefMax=[]  ReciprocalOutMin=[]  ReciprocalOutMax=[]  SumDenOutMin=[]  SumDenOutMax=[]  SumNumOutMin=[]  SumNumOutMax=[]  DivideOutMin=[]  DivideOutMax=[]  UdiffTsProdOutMin=[]  UdiffTsProdOutMax=[]  NTsProdOutMin=[]  NTsProdOutMax=[]  UintegralTsProdOutMin=[]  UintegralTsProdOutMax=[]  UngainTsProdOutMin=[]  UngainTsProdOutMax=[]  ClampingZeroOutDataTypeStr=Inherit: Inherit via back propagation  ClampingZeroOutMin=[]  ClampingZeroOutMax=[]  FilterDenConstantOutDataTypeStr=Inherit: Inherit via back propagation  FilterDenConstantOutMin=[]  FilterDenConstantOutMax=[]  PCopyOutDataTypeStr=Inherit: Inherit via back propagation  PCopyOutMin=[]  PCopyOutMax=[]  NCopyOutDataTypeStr=Inherit: Inherit via back propagation  NCopyOutMin=[]  NCopyOutMax=[]  IntegratorContinuousStateAttributes=''  IntegratorStateMustResolveToSignalObject=off  IntegratorRTWStateStorageClass=Auto  FilterContinuousStateAttributes=''  FilterStateMustResolveToSignalObject=off  FilterRTWStateStorageClass=Auto  ParallelPVariant=InternalParameters  IdealPVariant=Disabled  IVariant=InternalParameters  DVariant=Disabled  IntegratorVariant=Discrete  SatVariant=Disabled  AWVariant=Passthrough  PCopyVariant=Disabled  TRVariant=Disabled  FdbkBlocksVariant=Forward  IdealPFdbkVariant=Disabled  SatFdbkVariant=Disabled  DerivativeFilterVariant=Disabled  NVariant=Disabled  NCopyVariant=Disabled_SignalSpec  FilterICVariant=Disabled  IntegratorICVariant=InternalICs  ExternalResetVariant=Disabled  TRSumVariant=Passthrough  SumFdbkVariant=Disabled  SumVariant=Sum_PI  TsampFilterVariant=InternalTs  TsampNgainVariant=Passthrough  TsampIntegralVariant=Passthrough  ExternalSaturationOutDataTypeStr=Inherit: Same as second input
  rollrate_setpoint : Outport
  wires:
  roll_angle/1 -> Discrete D Controller/1
  roll_error/1 -> Discrete PI Controller/1
  Discrete PI Controller/1 -> Add/1
  Discrete D Controller/1 -> Add/2
  Add/1 -> rollrate_setpoint/1

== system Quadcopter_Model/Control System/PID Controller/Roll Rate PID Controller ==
  rollrate_error : Inport
  rollrate : Inport  Port=2
  Add : Sum  Inputs=+-
  Discrete D Controller : Derivative/Discrete D Controller  Kd=Kd  a=a
  Discrete PI Controller : slpidlib/PID Controller  Controller=PI  Form=Parallel  TimeDomain=Discrete-time  UseExternalTs=off  SampleTime=Ts  IntegratorMethod=Forward Euler  FilterMethod=Forward Euler  ControllerParametersSource=internal  P=Kp  I=Ki  UseKiTs=off  D=0  N=100  UseFilter=on  TunerSelectOption=Transfer Function Based (PID Tuner App)  InitialConditionSource=internal  InitialConditionForIntegrator=0  InitialConditionForFilter=0  DifferentiatorICPrevScaledInput=0  ExternalReset=none  TrackingMode=off  Kt=1  LimitOutput=off  SatLimitsSource=internal  UpperSaturationLimit=inf  LowerSaturationLimit=-inf  LinearizeAsGain=off  AntiWindupMode=none  Kb=1  LimitIntegrator=off  UpperIntegratorSaturationLimit=inf  LowerIntegratorSaturationLimit=-inf  POutMin=[]  POutMax=[]  IOutMin=[]  IOutMax=[]  DOutMin=[]  DOutMax=[]  NOutMin=[]  NOutMax=[]  SumOutMin=[]  SumOutMax=[]  SaturationOutMin=[]  SaturationOutMax=[]  PParamMin=[]  PParamMax=[]  IParamMin=[]  IParamMax=[]  DParamMin=[]  DParamMax=[]  NParamMin=[]  NParamMax=[]  KbParamMin=[]  KbParamMax=[]  KtParamMin=[]  KtParamMax=[]  KbOutMin=[]  KbOutMax=[]  KtOutMin=[]  KtOutMax=[]  IntegratorOutMin=[]  IntegratorOutMax=[]  FilterOutMin=[]  FilterOutMax=[]  SumI1OutMin=[]  SumI1OutMax=[]  SumI2OutMin=[]  SumI2OutMax=[]  SumI3OutMin=[]  SumI3OutMax=[]  SumI4OutMin=[]  SumI4OutMax=[]  SumDOutMin=[]  SumDOutMax=[]  DifferentiatorOutMin=[]  DifferentiatorOutMax=[]  FilterDiffOutCoefMin=[]  FilterDiffOutCoefMax=[]  ReciprocalOutMin=[]  ReciprocalOutMax=[]  SumDenOutMin=[]  SumDenOutMax=[]  SumNumOutMin=[]  SumNumOutMax=[]  DivideOutMin=[]  DivideOutMax=[]  UdiffTsProdOutMin=[]  UdiffTsProdOutMax=[]  NTsProdOutMin=[]  NTsProdOutMax=[]  UintegralTsProdOutMin=[]  UintegralTsProdOutMax=[]  UngainTsProdOutMin=[]  UngainTsProdOutMax=[]  ClampingZeroOutDataTypeStr=Inherit: Inherit via back propagation  ClampingZeroOutMin=[]  ClampingZeroOutMax=[]  FilterDenConstantOutDataTypeStr=Inherit: Inherit via back propagation  FilterDenConstantOutMin=[]  FilterDenConstantOutMax=[]  PCopyOutDataTypeStr=Inherit: Inherit via back propagation  PCopyOutMin=[]  PCopyOutMax=[]  NCopyOutDataTypeStr=Inherit: Inherit via back propagation  NCopyOutMin=[]  NCopyOutMax=[]  IntegratorContinuousStateAttributes=''  IntegratorStateMustResolveToSignalObject=off  IntegratorRTWStateStorageClass=Auto  FilterContinuousStateAttributes=''  FilterStateMustResolveToSignalObject=off  FilterRTWStateStorageClass=Auto  ParallelPVariant=InternalParameters  IdealPVariant=Disabled  IVariant=InternalParameters  DVariant=Disabled  IntegratorVariant=Discrete  SatVariant=Disabled  AWVariant=Passthrough  PCopyVariant=Disabled  TRVariant=Disabled  FdbkBlocksVariant=Forward  IdealPFdbkVariant=Disabled  SatFdbkVariant=Disabled  DerivativeFilterVariant=Disabled  NVariant=Disabled  NCopyVariant=Disabled_SignalSpec  FilterICVariant=Disabled  IntegratorICVariant=InternalICs  ExternalResetVariant=Disabled  TRSumVariant=Passthrough  SumFdbkVariant=Disabled  SumVariant=Sum_PI  TsampFilterVariant=InternalTs  TsampNgainVariant=Passthrough  TsampIntegralVariant=Passthrough  ExternalSaturationOutDataTypeStr=Inherit: Same as second input
  y_motor_command : Outport
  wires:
  rollrate/1 -> Discrete D Controller/1
  rollrate_error/1 -> Discrete PI Controller/1
  Discrete PI Controller/1 -> Add/1
  Discrete D Controller/1 -> Add/2
  Add/1 -> y_motor_command/1
